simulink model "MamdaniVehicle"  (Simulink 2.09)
settings: Solver=ode45  StartTime=0.0  StopTime=50  MaxStep=10  RelTol=1e-3  AbsTol=1e-3
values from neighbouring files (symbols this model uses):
  vd = 45    [VdataM.m]
undefined symbols (not defined in the file or in its folder): sfunyst
libraries: fuzzy x4

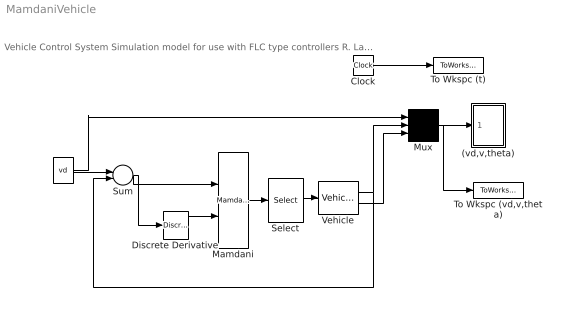
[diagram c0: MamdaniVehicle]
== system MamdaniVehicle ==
  note: Vehicle Control System Simulation model for use with FLC type controllers R. Langari 3/1/97
  " " : Constant  Value=vd
  (vd,v,theta) : Subsystem  mask(Storage scope.){}
      mask help: Storage scope using MATLAB graph window. Enter plotting ranges and line type.
      mask init:
      | npts = @4; color = @5; ax = [0, @1, @2, @3]; dt=-1;
  Clock : Clock
  Discrete Derivative : fuzzy/Discrete Derivative
  Mamdani : fuzzy/Mamdani
  Mux : Mux  Inputs=3
  Select : fuzzy/Select
  Sum : Sum  Inputs=+-
  To Wkspc (vd,v,theta) : ToWorkspace  VariableName=yout  SampleTime=0
  To Wkspc (t) : ToWorkspace  VariableName=t  SampleTime=0
  Vehicle : fuzzy/Vehicle
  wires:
  Select/1 -> Vehicle/1
  Clock/1 -> To Wkspc (t)/1
  Sum/1 -> Mamdani/1, Discrete Derivative/1
  Discrete Derivative/1 -> Mamdani/2
  " "/1 -> Sum/1, Mux/1
  Mamdani/1 -> Select/1
  Vehicle/2 -> Mux/3
  Vehicle/1 -> Mux/2, Sum/2
  Mux/1 -> To Wkspc (vd,v,theta)/1, (vd,v,theta)/1(x)

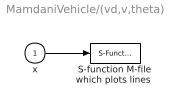
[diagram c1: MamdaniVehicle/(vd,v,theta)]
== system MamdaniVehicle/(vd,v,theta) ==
  x : Inport  Port=1  PortWidth=-1  SampleTime=-1
  "S-function M-file which plots lines " : S-Function  LoadFcn=sfunyst([],[],[],'LoadBlock')  FunctionName=sfunyst  Parameters=ax, color, npts, dt
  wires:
  x/1 -> "S-function M-file which plots lines "/1
